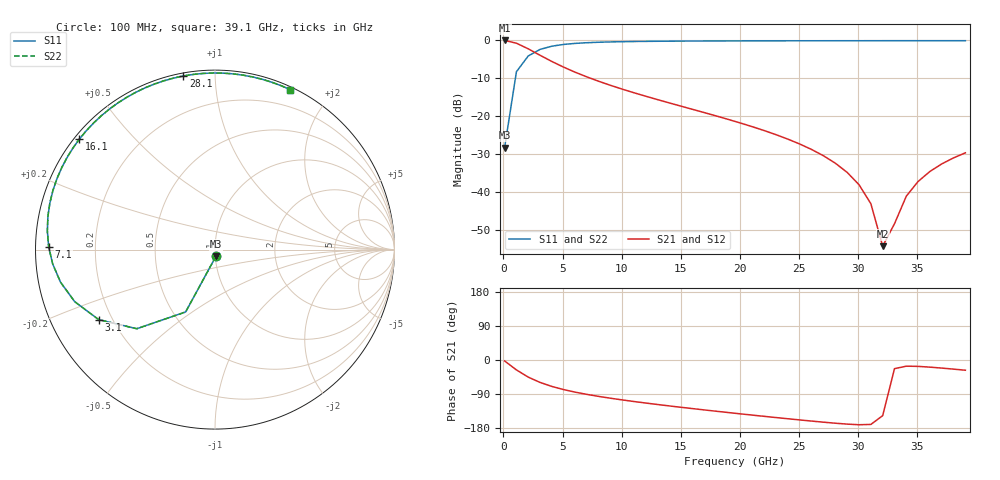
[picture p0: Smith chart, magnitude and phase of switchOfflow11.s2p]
# GHZ S RI R 50
!Output file by Shape3_29
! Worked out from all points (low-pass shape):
!   40 points, 100 MHz to 39.1 GHz, reference 50 ohm
!   highest |S21| = -0.07 dB at 100 MHz (marker M1); lowest = -54.3 dB at 32.1 GHz (marker M2)
!   |S21| within 3 dB of the highest: start of sweep to 2.567 GHz
!   lowest |S11| = -28.3 dB at 100 MHz (marker M3), VSWR 1.08, Z = 50.3 - j3.83 ohm
!   |S11| at or under -10 dB: start of sweep to 1.016 GHz
!   |S22| runs from -28.3 to -0.1 dB; largest |S21 - S12| = 1.1e-13
!   S11 on the Smith chart (normalised r, x): 100 MHz: 1.01, -0.08; 3.1 GHz: 0.15, -0.27; 7.1 GHz: 0.04, +0.01; 16.1 GHz: 0.01, +0.36; 28.1 GHz: 0.01, +0.83; 39.1 GHz: 0.03, +1.58
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0.1  0.00479 -0.038  0.9911 -0.0434  0.9911 -0.0434  0.00479 -0.038
1.1  -0.1637 -0.3474  0.8195 -0.4029  0.8195 -0.4029  -0.1637 -0.3474
2.1  -0.4358 -0.4408  0.5428 -0.5453  0.5428 -0.5453  -0.4358 -0.4409
3.1  -0.6477 -0.3902  0.3241 -0.5434  0.3241 -0.5434  -0.6477 -0.3903
4.1  -0.7815 -0.2901  0.1812 -0.4916  0.1812 -0.4916  -0.7815 -0.2902
5.1  -0.8604 -0.1819  0.0909 -0.4313  0.0909 -0.4313  -0.8605 -0.182
7.1  -0.9268 0.0167  -0.00535 -0.3263  -0.00535 -0.3263  -0.9269 0.0167
10.1  -0.9199 0.26  -0.0603 -0.217  -0.0603 -0.217  -0.92 0.26
13.1  -0.8545 0.4555  -0.076 -0.145  -0.076 -0.145  -0.8545 0.4555
16.1  -0.7553 0.6159  -0.0758 -0.0949  -0.0758 -0.0949  -0.7554 0.6159
20.1  -0.5873 0.7835  -0.0637 -0.0493  -0.0637 -0.0493  -0.5873 0.7835
23.1  -0.4418 0.8761  -0.0499 -0.0266  -0.0499 -0.0266  -0.4418 0.8762
26.1  -0.2847 0.9404  -0.0342 -0.0116  -0.0342 -0.0116  -0.2848 0.9405
28.1  -0.1758 0.9674  -0.0232 -0.00543  -0.0232 -0.00543  -0.1759 0.9675
30.1  -0.0651 0.9816  -0.0123 -0.00198  -0.0123 -0.00198  -0.0651 0.9817
31.1  -0.00942 0.9839  -0.00688 -0.00121  -0.00688 -0.00121  -0.00948 0.984
32.1  0.0462 0.9831  -0.00161 -0.00105  -0.00161 -0.00105  0.0461 0.9831
33.1  0.1015 0.9791  0.0035 -0.00148  0.0035 -0.00148  0.1015 0.9791
34.1  0.1565 0.9719  0.00843 -0.00246  0.00843 -0.00246  0.1565 0.972
35.1  0.211 0.9617  0.0131 -0.00398  0.0131 -0.00398  0.2109 0.9618
37.1  0.3176 0.9321  0.0218 -0.00851  0.0218 -0.00851  0.3175 0.9322
39.1  0.4201 0.8907  0.0292 -0.0149  0.0292 -0.0149  0.42 0.8908
